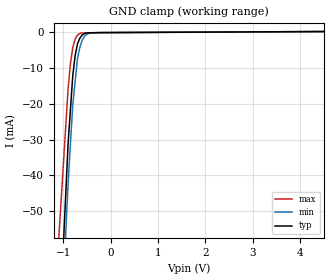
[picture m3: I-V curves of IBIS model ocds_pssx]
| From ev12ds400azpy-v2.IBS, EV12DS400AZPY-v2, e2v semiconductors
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[Model] ocds_pssx
Model_type Input
Vinl = 800.000mV
Vinh = 1.60000V
C_comp 578.000fF 540.000fF 616.000fF
| variable typ   min   max
[Voltage Range] 3.30000V 3.15000V 3.45000V
[POWER Clamp Reference] 3.30000V 3.15000V 3.45000V
[GND Clamp Reference] 0.00000V 0.00000V 0.00000V
[Temperature Range]   25   110   -40
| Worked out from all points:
|   GND clamp passes 1 mA (typ) near -0.61 V on its own axis
[GND Clamp]
-3.3V     -719.1mA   -732.9mA   -525.7mA
-900mV    -31.45mA   -42.54mA   -16.04mA
-850mV    -21.81mA   -31.45mA   -8.854mA
-800mV    -12.16mA   -20.36mA   -4.345mA
-750mV    -6.542mA   -13.84mA   -1.89mA
-700mV    -3.28mA    -7.322mA   -781.2uA
-650mV    -1.67mA    -4.224mA   -365.4uA
-600mV    -773.9uA   -2.19mA    -196.8uA
-550mV    -373.1uA   -1.098mA   -184.9uA
-500mV    -211.1uA   -559.7uA   -173.1uA
-400mV    -175.4uA   -185.3uA   -149.3uA
6.6V      319uA      321.4uA    307.8uA
[POWER Clamp]
-3.3V     0A         0A         0A
6.6V      0A         0A         0A
